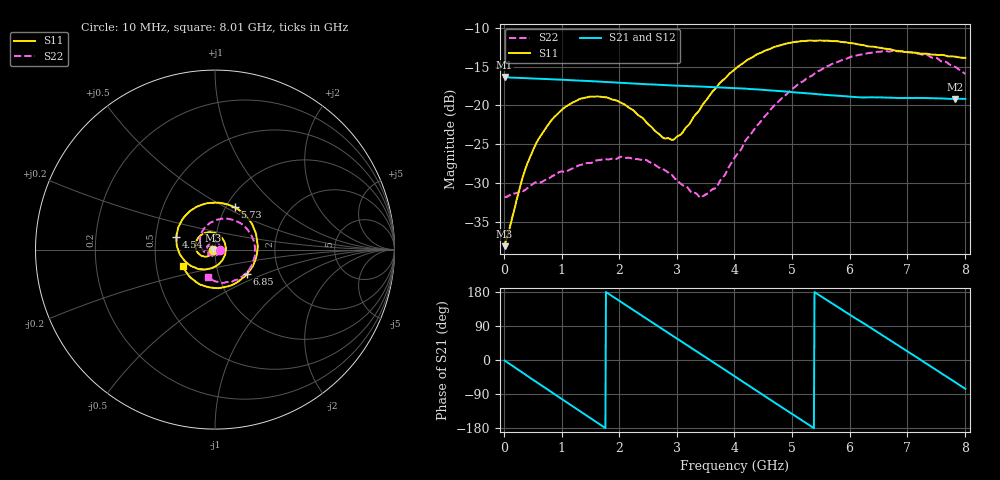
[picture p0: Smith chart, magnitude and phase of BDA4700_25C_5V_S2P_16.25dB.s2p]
!Agilent Technologies,E5071B,MY42404982,A.09.10
!Date: Mon Oct 20 13:34:23 2025
!Data & Calibration Information:
!Freq	S11:SOLT2(ON)	S21:SOLT2(ON)	S12:SOLT2(ON)	S22:SOLT2(ON)
# Hz S RI R 50
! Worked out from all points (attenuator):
!   801 points, 10 MHz to 8.01 GHz, reference 50 ohm
!   highest |S21| = -16.35 dB at 10 MHz (marker M1); lowest = -19.2 dB at 7.83 GHz (marker M2)
!   lowest |S11| = -38.1 dB at 10 MHz (marker M3), VSWR 1.03, Z = 48.8 - j0.164 ohm
!   |S11| at or under -10 dB: start of sweep to end of sweep
!   |S22| runs from -31.9 to -13.0 dB; largest |S21 - S12| = 0.0012
!   S11 on the Smith chart (normalised r, x): 10 MHz: 0.98, -0.00; 4.54 GHz: 0.64, +0.09; 5.73 GHz: 1.10, +0.56; 6.85 GHz: 1.37, -0.39; 8.01 GHz: 0.68, -0.13
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1e7  -0.0123 -0.00168  0.1523 -0.00328  0.1523 -0.00344  0.0257 -0.000866
3.4e8  -0.0238 -0.0271  0.1224 -0.0868  0.1223 -0.087  0.0224 -0.0174
5.6e8  -0.0425 -0.0383  0.0792 -0.126  0.0791 -0.1262  0.0146 -0.0284
8.8e8  -0.0781 -0.0332  -0.00135 -0.1471  -0.00137 -0.1473  -0.00766 -0.0349
1.35e9  -0.1092 0.0207  -0.1076 -0.0961  -0.1077 -0.0962  -0.038 -0.0168
1.97e9  -0.0504 0.0943  -0.1312 0.0498  -0.1313 0.0498  -0.0329 0.0315
2.45e9  0.0297 0.0738  -0.0499 0.1277  -0.0499 0.1278  0.00176 0.0447
2.68e9  0.0545 0.037  0.00362 0.1358  0.00352 0.1359  0.0178 0.0358
2.96e9  0.0575 -0.0198  0.0655 0.1171  0.0656 0.117  0.0288 0.0184
3.43e9  -0.00815 -0.0983  0.1283 0.0323  0.1283 0.0323  0.0177 -0.0184
3.69e9  -0.0718 -0.1097  0.1281 -0.0264  0.1282 -0.0268  -0.00318 -0.0296
4.01e9  -0.1527 -0.0773  0.0938 -0.0893  0.0939 -0.0892  -0.0374 -0.0275
4.54e9  -0.2153 0.0686  -0.0145 -0.1248  -0.0144 -0.125  -0.0812 0.0288
4.9e9  -0.1713 0.1823  -0.0829 -0.0908  -0.0827 -0.0911  -0.0759 0.0899
5.35e9  -0.0317 0.2596  -0.1189 -0.00658  -0.1188 -0.00692  -0.013 0.1552
5.73e9  0.1097 0.2354  -0.0962 0.0648  -0.0961 0.0648  0.0744 0.1714
6.21e9  0.2252 0.0972  -0.0194 0.1109  -0.0184 0.1113  0.1822 0.1104
6.68e9  0.2162 -0.0808  0.0656 0.091  0.0658 0.091  0.2221 -0.0108
6.85e9  0.1786 -0.1359  0.0882 0.0683  0.0885 0.0679  0.215 -0.0585
7.33e9  0.0184 -0.2147  0.1102 -0.0177  0.1102 -0.0179  0.1347 -0.1631
7.83e9  -0.1463 -0.1459  0.058 -0.0936  0.058 -0.0938  0.00248 -0.1774
8.01e9  -0.1806 -0.0922  0.0262 -0.1071  0.0263 -0.1072  -0.0396 -0.1544
